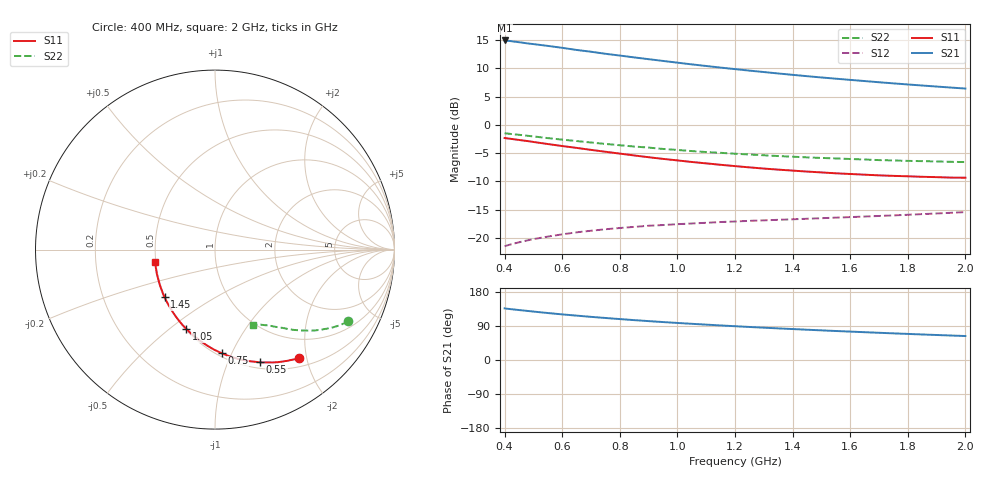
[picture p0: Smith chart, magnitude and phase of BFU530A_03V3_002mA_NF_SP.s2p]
! Filename:  P:\Prog\Test\Noise\ATS_data\Testdata_Net\06 Compressed Noise after Statistics\BFU530A_APG2013_33_A05_03p3V_002mA_SP_CM01_D.sf
! Date/Time: Tue 16/Apr/2013 15:10:57
! BFU530A_APG2013_33_A05_03p3V_1to25mA_NF_CM01_Bias2_R.sf
! Noise Parameter Data File
! BFU530A_APG2013_33_A05_03p3V_1to25mA_NF_CM01
! Date/time: Fri Apr 12 14:21:19 2013
! VAR V_out= 3.301000
! VAR I_out= 2.000000
! VAR V_in= 0.801400
! VAR I_in= 0.021200
! Device data file deembeded for feedlines and parallel
! Original file: \06 Compressed Noise after Statistics\BFU530A_APG2013_33_A05_03p3V_002mA_SP_CM01_R.sf
! Feed-files: PR017V01_150413_Feed1.s2p, PR017V01_150413_Feed2.s2p
! Parallel-file: PR017V01_150413_Par.s2p
# MHz S MA R 50
!  Freq-MHz  S11-mag  S11-arg  S21-mag  S21-arg  S12-mag  S12-arg  S22-mag  S22-arg
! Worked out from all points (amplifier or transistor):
!   37 points, 400 MHz to 2 GHz, reference 50 ohm
!   highest |S21| = 14.9 dB at 400 MHz (marker M1)
!   |S21| within 3 dB of that: start of sweep to 851 MHz
!   unconditionally stable (mu >= 1): nowhere
!   at 500 MHz: K = 0.34, MSG = 17.2 dB, |S12| = -20.2 dB
!   at 1.1 GHz: K = 0.68, MSG = 13.9 dB, |S12| = -17.3 dB
!   at 2 GHz: K = 1.00, MSG = 10.9 dB, |S12| = -15.4 dB
!   lowest NFmin = 0.47 dB at 433 MHz
!   S11 on the Smith chart (normalised r, x): 400 MHz: 0.64, -1.87; 550 MHz: 0.57, -1.32; 750 MHz: 0.53, -0.92; 1.05 GHz: 0.51, -0.57; 1.45 GHz: 0.50, -0.31; 2 GHz: 0.50, -0.08
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400  0.7648 -52.0  5.564 136.2  0.08474 61.1  0.8425 -28.4
420  0.7529 -54.4  5.495 134.3  0.08764 60.1  0.8316 -29.4
460  0.7293 -58.7  5.328 131.0  0.093 58.2  0.8115 -31.4
500  0.7059 -63.0  5.168 127.8  0.09781 56.5  0.7901 -33.1
550  0.6767 -68.2  4.981 124.0  0.103 54.5  0.7634 -35.2
600  0.6496 -73.0  4.789 120.4  0.1078 52.9  0.7399 -37.1
650  0.6256 -77.5  4.587 117.1  0.1123 51.4  0.7193 -38.7
700  0.6008 -82.1  4.424 113.8  0.1159 50.1  0.6975 -40.4
750  0.5784 -86.3  4.243 110.9  0.1195 49.0  0.6783 -41.7
850  0.5363 -94.7  3.942 105.2  0.1255 47.1  0.643 -44.3
900  0.5174 -98.7  3.801 102.6  0.1284 46.3  0.6293 -45.4
950  0.5003 -102.5  3.669 100.1  0.1302 45.8  0.6126 -46.5
1050  0.4698 -109.8  3.42 95.5  0.1344 45.0  0.5863 -48.4
1150  0.4436 -117.0  3.204 91.2  0.1385 44.4  0.5659 -50.2
1200  0.4318 -120.4  3.106 89.2  0.14 44.3  0.5553 -51.1
1300  0.4109 -127.0  2.927 85.3  0.1433 44.3  0.5385 -52.7
1450  0.3865 -136.6  2.691 79.9  0.148 44.7  0.516 -55.0
1500  0.3799 -139.8  2.62 78.2  0.1497 44.9  0.51 -55.8
1650  0.3628 -148.7  2.436 73.4  0.1548 45.9  0.494 -58.1
1750  0.3541 -154.5  2.324 70.3  0.1585 46.8  0.4845 -59.5
1850  0.3475 -160.0  2.225 67.4  0.1626 47.6  0.4779 -61.0
2000  0.341 -168.0  2.092 63.2  0.1695 49.0  0.4687 -63.4
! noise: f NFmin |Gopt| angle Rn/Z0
400  0.5238  0.4882  22.34  0.1975
460  0.5248  0.4852  29.23  0.1885
600  0.5974  0.4754  34.96  0.1956
800  0.6009  0.4463  52.94  0.156
1000  0.6595  0.4226  64.61  0.1435
1200  0.7077  0.4114  78.34  0.1395
1400  0.7153  0.3939  90.54  0.1262
1600  0.8033  0.3863  107.2  0.0968
1800  0.8163  0.3832  117.9  0.0814
2000  0.8074  0.3885  138.6  0.0665
